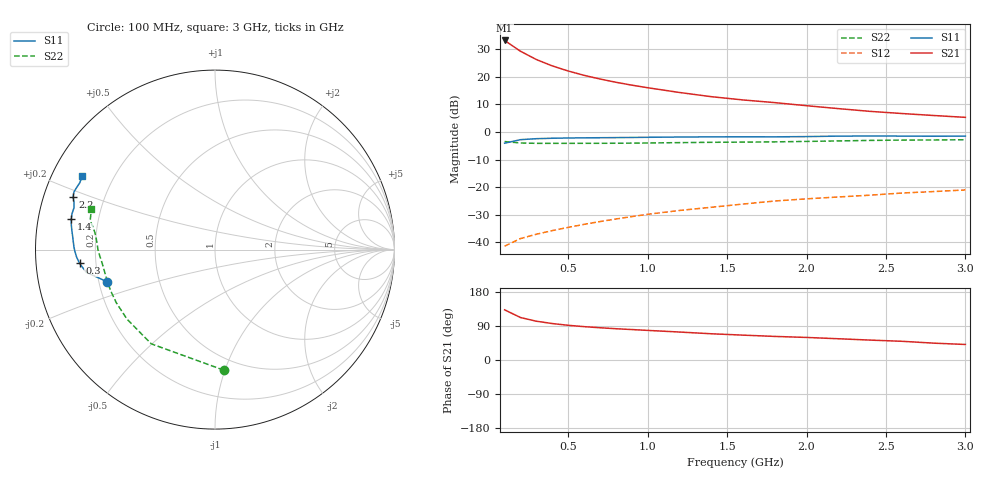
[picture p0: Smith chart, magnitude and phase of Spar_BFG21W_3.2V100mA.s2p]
! Filename: 3_2100bfg21.001
! Title: BFG21W
! Bias: Vce=3.2V; Ic=100mA
! Company: NXP Semiconductors NL
! User: Quality&Reliability T&D
! Measure time: 10 Nov 1999 / 11:42:53
#  MHz  S  MA  R 50
! Freq  S11  S21  S12  S22  :
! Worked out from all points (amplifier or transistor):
!   20 points, 100 MHz to 3 GHz, reference 50 ohm
!   highest |S21| = 33.2 dB at 100 MHz (marker M1)
!   |S21| within 3 dB of that: start of sweep to 176.6 MHz
!   unconditionally stable (mu >= 1): 687.4 MHz to end of sweep
!   at 400 MHz: K = 0.86, MSG = 29.9 dB, |S12| = -35.7 dB
!   at 1.2 GHz: K = 1.06, MAG = 19.9 dB, |S12| = -28.4 dB
!   at 3 GHz: K = 1.05, MAG = 11.8 dB, |S12| = -21.0 dB
!   S11 on the Smith chart (normalised r, x): 100 MHz: 0.23, -0.14; 300 MHz: 0.14, -0.05; 1.4 GHz: 0.10, +0.10; 2.2 GHz: 0.09, +0.18; 3 GHz: 0.09, +0.26
100  0.6285 -163.5  45.73 132.4  0.008552 55.6  0.6733 -85.8
200  0.7281 -170.0  29.14 112.1  0.01175 51.0  0.6339 -124.1
300  0.7586 -174.2  20.62 102.3  0.01408 53.7  0.6249 -141.7
400  0.7726 -177.0  15.81 96.2  0.01635 57.3  0.6244 -151.6
500  0.7808 -179.3  12.78 91.6  0.01873 60.2  0.6248 -158.0
600  0.7861 178.9  10.67 88.0  0.02125 62.6  0.6255 -162.4
700  0.7898 177.2  9.16 85.1  0.02388 65.0  0.6259 -165.9
800  0.7938 175.6  7.994 82.5  0.02658 66.7  0.6273 -168.7
900  0.7984 174.1  7.088 80.4  0.02935 68.3  0.6301 -171.2
1000  0.8038 172.7  6.363 78.1  0.0323 69.2  0.634 -173.5
1200  0.8128 170.1  5.22 73.8  0.03794 70.6  0.6435 -177.0
1400  0.8187 168.0  4.381 69.2  0.04331 71.1  0.6522 -180.0
1600  0.8214 165.8  3.822 65.6  0.04956 71.5  0.657 177.4
1800  0.8193 163.4  3.417 62.2  0.05629 71.7  0.6647 174.7
2000  0.828 161.5  3.005 59.5  0.06165 72.2  0.6763 171.9
2200  0.8438 159.6  2.661 56.1  0.0666 72.1  0.691 169.6
2400  0.8487 157.8  2.372 52.5  0.07181 71.3  0.7056 167.8
2600  0.8453 156.0  2.169 49.4  0.07855 70.3  0.7149 166.3
2800  0.8405 153.7  1.997 44.5  0.08349 68.6  0.719 164.2
3000  0.8448 151.1  1.847 41.0  0.08939 67.7  0.7261 161.7
